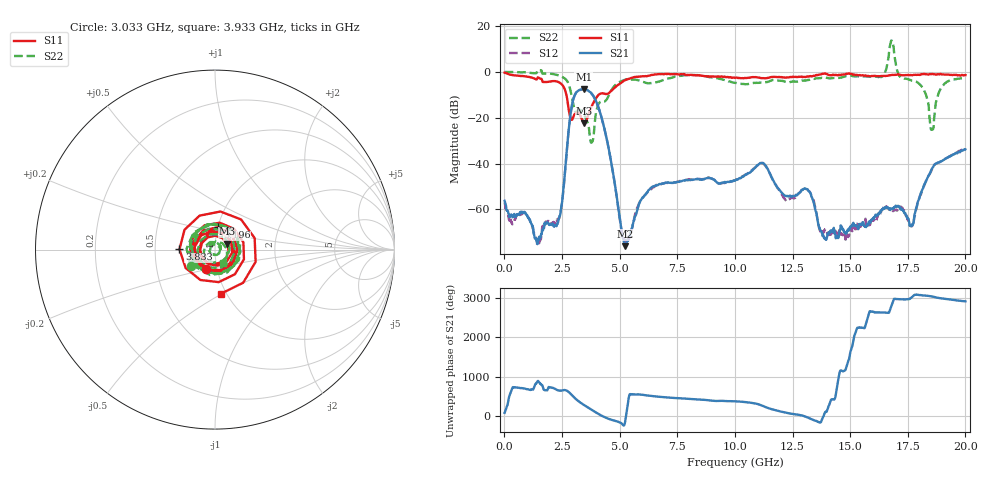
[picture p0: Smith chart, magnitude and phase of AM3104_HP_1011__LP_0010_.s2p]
!Created with skrf (http://scikit-rf.org).
# Hz S RI R 50.0
!freq ReS11 ImS11 ReS21 ImS21 ReS12 ImS12 ReS22 ImS22
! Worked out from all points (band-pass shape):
!   1601 points, 10 MHz to 20 GHz, reference 50 ohm
!   highest |S21| = -7.59 dB at 3.446 GHz (marker M1); lowest = -76.0 dB at 5.245 GHz (marker M2)
!   |S21| within 3 dB of the highest: 3.037 GHz to 3.864 GHz (827.5 MHz wide, 24 % of centre)
!   lowest |S11| = -22.4 dB at 3.471 GHz (marker M3), VSWR 1.16, Z = 57.2 + j3.75 ohm
!   |S11| at or under -10 dB: 2.689 GHz to 4.087 GHz (1.398 GHz wide, 41.3 % of centre)
!   |S22| runs from -30.9 to 13.7 dB; largest |S21 - S12| = 0.016
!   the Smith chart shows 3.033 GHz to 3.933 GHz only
!   S11 on the Smith chart (normalised r, x): 3.033 GHz: 0.89, -0.19; 3.196 GHz: 1.00, +0.25; 3.833 GHz: 0.67, +0.00; 3.933 GHz: 0.94, -0.49
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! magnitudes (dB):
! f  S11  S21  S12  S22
! 10 MHz  -0.3  -56.3  -57.0  -0.1
! 1.472 GHz  -2.5  -72.8  -75.8  0.8
! 2.246 GHz  -4.1  -67.2  -64.9  -1.3
! 3.033 GHz  -18.7  -10.7  -10.7  -15.7
! 3.196 GHz  -18.0  -8.3  -8.4  -16.8
! 3.346 GHz  -20.3  -7.7  -7.7  -16.9
! 3.446 GHz  -22.2  -7.6  -7.6  -18.6
! 3.471 GHz  -22.4  -7.6  -7.7  -19.0
! 3.833 GHz  -14.1  -10.1  -10.1  -30.1
! 3.933 GHz  -12.1  -11.8  -11.9  -21.1
! 5.245 GHz  -3.6  -76.0  -73.3  -3.4
! 6.682 GHz  -1.0  -49.2  -49.2  -4.3
! 10.01 GHz  -2.6  -47.5  -47.3  -4.8
! 11.19 GHz  -2.8  -39.8  -39.9  -4.6
! 12.2 GHz  -2.5  -54.1  -56.1  -4.3
! 13.34 GHz  -2.0  -54.8  -54.1  -3.3
! 13.9 GHz  -0.7  -72.3  -69.1  -2.4
! 16.68 GHz  -1.5  -59.6  -60.0  7.2
! 17.66 GHz  -1.5  -67.2  -67.2  -3.8
! 18.54 GHz  -0.9  -42.5  -42.7  -25.3
! 18.99 GHz  -1.1  -38.8  -38.7  -6.4
! 20 GHz  -1.4  -33.8  -33.4  -2.5
